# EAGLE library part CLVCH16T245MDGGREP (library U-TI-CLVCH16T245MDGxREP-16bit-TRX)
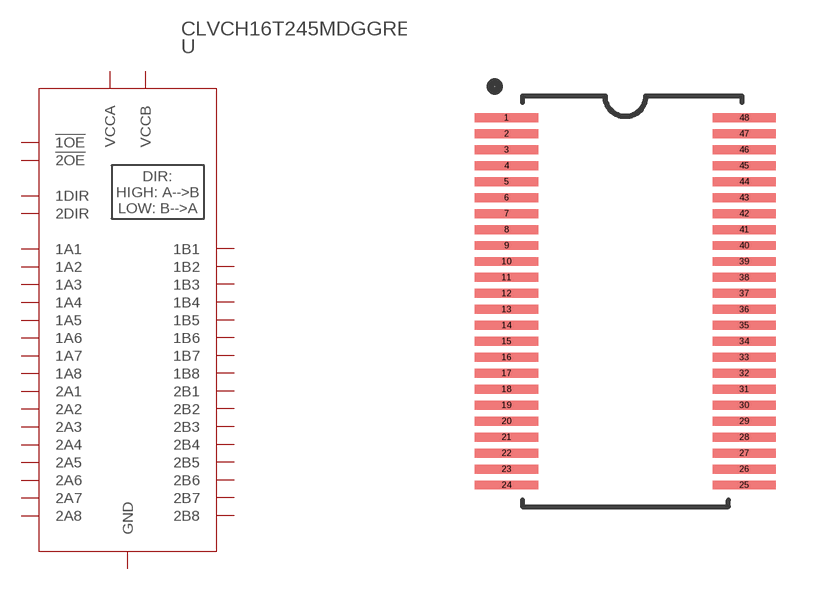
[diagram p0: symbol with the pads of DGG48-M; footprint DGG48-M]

Designator prefix U

## CLVCH16T245MDGGREP  [DGG48-M]
1  1DIR  in
2  1B1
3  1B2
4  GND  pwr
5  1B3
6  1B4
7  VCCB  pwr
8  1B5
9  1B6
10  GND  pwr
11  1B7
12  1B8
13  2B1
14  2B2
15  GND  pwr
16  2B3
17  2B4
18  VCCB  pwr
19  2B5
20  2B6
21  GND  pwr
22  2B7
23  2B8
24  2DIR  in
25  !2OE  in
26  2A8
27  2A7
28  GND  pwr
29  2A6
30  2A5
31  VCCA  pwr
32  2A4
33  2A3
34  GND  pwr
35  2A2
36  2A1
37  1A8
38  1A7
39  GND  pwr
40  1A6
41  1A5
42  VCCA  pwr
43  1A4
44  1A3
45  GND  pwr
46  1A2
47  1A1
48  !1OE  in

## Footprint DGG48-M (pad centres in mm)
smd 1.981 x 0.279: 1 -3.721,5.75; 2 -3.721,5.25; 3 -3.721,4.75; 4 -3.721,4.25; 5 -3.721,3.75; 6 -3.721,3.25; 7 -3.721,2.75; 8 -3.721,2.25; 9 -3.721,1.75; 10 -3.721,1.25; 11 -3.721,0.75; 12 -3.721,0.25; 13 -3.721,-0.25; 14 -3.721,-0.75; 15 -3.721,-1.25; 16 -3.721,-1.75; 17 -3.721,-2.25; 18 -3.721,-2.75; 19 -3.721,-3.25; 20 -3.721,-3.75; 21 -3.721,-4.25; 22 -3.721,-4.75; 23 -3.721,-5.25; 24 -3.721,-5.75; 25 3.721,-5.75; 26 3.721,-5.25; 27 3.721,-4.75; 28 3.721,-4.25; 29 3.721,-3.75; 30 3.721,-3.25; 31 3.721,-2.75; 32 3.721,-2.25; 33 3.721,-1.75; 34 3.721,-1.25; 35 3.721,-0.75; 36 3.721,-0.25; 37 3.721,0.25; 38 3.721,0.75; 39 3.721,1.25; 40 3.721,1.75; 41 3.721,2.25; 42 3.721,2.75; 43 3.721,3.25; 44 3.721,3.75; 45 3.721,4.25; 46 3.721,4.75; 47 3.721,5.25; 48 3.721,5.75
